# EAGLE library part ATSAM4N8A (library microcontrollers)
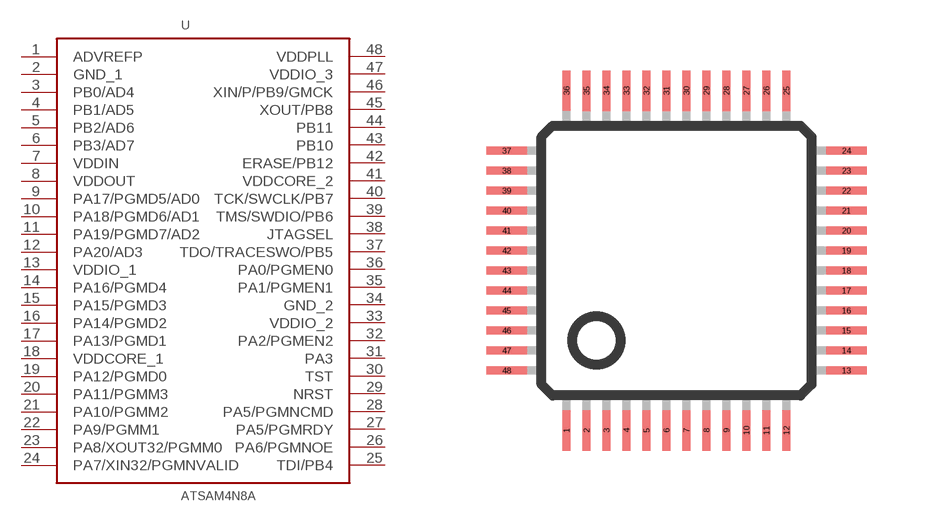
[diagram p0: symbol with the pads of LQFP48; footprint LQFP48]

Designator prefix U

## ATSAM4N8AATSAM4N8A  [LQFP48]
1  ADVREFP
2  GND_1
3  PB0/AD4
4  PB1/AD5
5  PB2/AD6
6  PB3/AD7
7  VDDIN
8  VDDOUT
9  PA17/PGMD5/AD0
10  PA18/PGMD6/AD1
11  PA19/PGMD7/AD2
12  PA20/AD3
13  VDDIO_1
14  PA16/PGMD4
15  PA15/PGMD3
16  PA14/PGMD2
17  PA13/PGMD1
18  VDDCORE_1
19  PA12/PGMD0
20  PA11/PGMM3
21  PA10/PGMM2
22  PA9/PGMM1
23  PA8/XOUT32/PGMM0
24  PA7/XIN32/PGMNVALID
25  TDI/PB4
26  PA6/PGMNOE
27  PA5/PGMRDY
28  PA5/PGMNCMD
29  NRST
30  TST
31  PA3
32  PA2/PGMEN2
33  VDDIO_2
34  GND_2
35  PA1/PGMEN1
36  PA0/PGMEN0
37  TDO/TRACESWO/PB5
38  JTAGSEL
39  TMS/SWDIO/PB6
40  TCK/SWCLK/PB7
41  VDDCORE_2
42  ERASE/PB12
43  PB10
44  PB11
45  XOUT/PB8
46  XIN/P/PB9/GMCK
47  VDDIO_3
48  VDDPLL

## Footprint LQFP48 (pad centres in mm)
48-pin plastic LQFP (FPT-48P-M26) www.fma.fujitsu.com/pdf/e713717.pdf
smd 0.203 x 1.016: 1 -2.75,-4.25; 2 -2.25,-4.25; 3 -1.75,-4.25; 4 -1.25,-4.25; 5 -0.75,-4.25; 6 -0.25,-4.25; 7 0.25,-4.25; 8 0.75,-4.25; 9 1.25,-4.25; 10 1.75,-4.25; 11 2.25,-4.25; 12 2.75,-4.25; 25 2.75,4.25; 26 2.25,4.25; 27 1.75,4.25; 28 1.25,4.25; 29 0.75,4.25; 30 0.25,4.25; 31 -0.25,4.25; 32 -0.75,4.25; 33 -1.25,4.25; 34 -1.75,4.25; 35 -2.25,4.25
smd 1.016 x 0.203: 13 4.25,-2.75; 14 4.25,-2.25; 15 4.25,-1.75; 16 4.25,-1.25; 17 4.25,-0.75; 18 4.25,-0.25; 19 4.25,0.25; 20 4.25,0.75; 21 4.25,1.25; 22 4.25,1.75; 23 4.25,2.25; 24 4.25,2.75; 37 -4.25,2.75; 38 -4.25,2.25; 39 -4.25,1.75; 40 -4.25,1.25; 41 -4.25,0.75; 42 -4.25,0.25; 43 -4.25,-0.25; 44 -4.25,-0.75; 45 -4.25,-1.25; 46 -4.25,-1.75; 47 -4.25,-2.25; 48 -4.25,-2.75
smd 0.203 x 1: 36 -2.75,4.25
